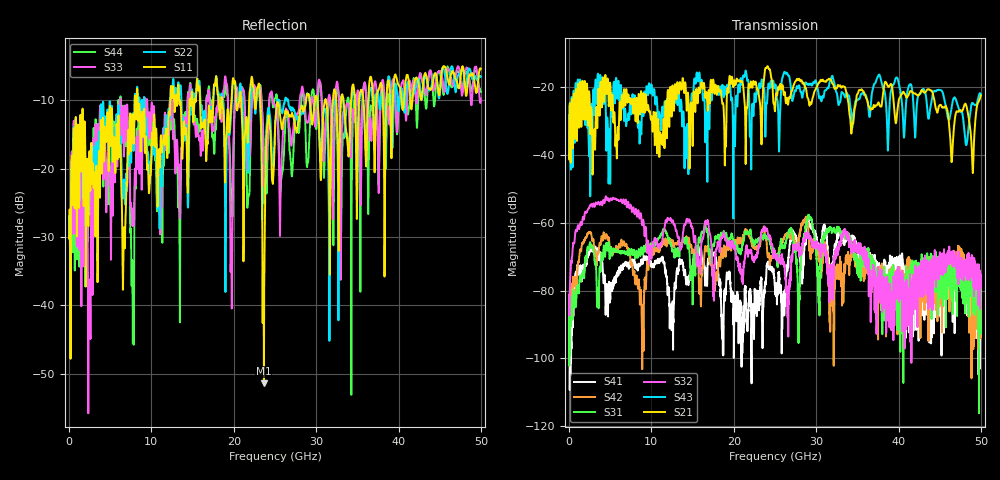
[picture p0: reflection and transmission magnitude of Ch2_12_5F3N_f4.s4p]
!Agilent Technologies,N5247A,US51170199,A.09.90.13
!Agilent N5247A: A.09.90.13
!Date: Tuesday, December 08, 2015 12:36:31
!Correction: S11(Full 4 Port(1,2,3,4))
!S12(Full 4 Port(1,2,3,4))
!S13(Full 4 Port(1,2,3,4))
!S14(Full 4 Port(1,2,3,4))
!S21(Full 4 Port(1,2,3,4))
!S22(Full 4 Port(1,2,3,4))
!S23(Full 4 Port(1,2,3,4))
!S24(Full 4 Port(1,2,3,4))
!S31(Full 4 Port(1,2,3,4))
!S32(Full 4 Port(1,2,3,4))
!S33(Full 4 Port(1,2,3,4))
!S34(Full 4 Port(1,2,3,4))
!S41(Full 4 Port(1,2,3,4))
!S42(Full 4 Port(1,2,3,4))
!S43(Full 4 Port(1,2,3,4))
!S44(Full 4 Port(1,2,3,4))
!S4P File: Measurements: <S11,S12,S13,S14>,
!<S21,S22,S23,S24>,
!<S31,S32,S33,S34>,
!<S41,S42,S43,S44>:
# Hz S  dB  R 50
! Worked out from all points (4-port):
!   3201 points, 10 MHz to 50 GHz, reference 50 ohm
!   strongest paths, dB at 10 MHz, 12.51 GHz, 25 GHz, 37.5 GHz, 50 GHz:
!     S21: -41.3, -21.6, -27.1, -24.7, -22.5
!     S43: -40.8, -22.7, -19.7, -16.9, -22.1
!     S32: -81.2, -59.5, -69.0, -79.8, -79.0
!     S31: -86.3, -68.0, -69.9, -73.2, -92.7
!     S42: -84.2, -66.5, -69.8, -82.4, -77.3
!     S41: -85.6, -84.0, -79.8, -73.2, -91.7
!   lowest |S11| = -51.4 dB at 23.66 GHz (marker M1), VSWR 1.01, Z = 50.2 - j0.123 ohm
!   |S11| at or under -10 dB: start of sweep to 7.975 GHz; 8.34 GHz to 12.29 GHz (3.948 GHz wide, 38.3 % of centre); 23.21 GHz to 28.79 GHz (5.583 GHz wide, 21.5 % of centre)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
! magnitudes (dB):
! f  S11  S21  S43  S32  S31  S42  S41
! 10 MHz  -30.2  -41.3  -40.8  -81.2  -86.3  -84.2  -85.6
! 4.603 GHz  -13.3  -19.8  -29.7  -53.3  -67.1  -64.0  -78.1
! 22.19 GHz  -6.6  -19.9  -27.5  -69.5  -65.1  -66.6  -92.4
! 23.66 GHz  -51.4  -17.8  -20.3  -61.3  -63.4  -61.2  -81.4
! 29.11 GHz  -9.2  -24.6  -19.1  -64.7  -57.7  -64.7  -59.6
! 30.32 GHz  -12.7  -18.6  -22.7  -67.8  -83.7  -69.2  -68.2
! 50 GHz  -5.4  -22.5  -22.1  -79.0  -92.7  -77.3  -91.7
